[IBIS VER]   5.0
[File Name]   f28p551pm.ibs
[File Rev]   1.0
[Date]   August 04, 2025
[Source]   File originated at Texas Instruments
[Copyright]   (c) 2012, Texas Instruments Inc.
[Component]   f28p551pm
[Manufacturer]  Texas Instruments
[Package]
| Variable   Typ   Min   Max
R_pkg  2.56E-01  1.11E-01  3.13E-01
L_pkg  6.62E-09  4.95E-09  7.77E-09
C_pkg  9.34E-15  7.88E-15  1.08E-14
[Pin]   signal_name   model_name   R_pin   L_pin   C_pin
   1   GPIO29   BCF3385DSHYPBFZ_LC  2.96E-01  7.53E-09  1.05E-14
   2   A16,B16,C16,GPIO28   BCF3385DSHYPBFZ_LC  2.80E-01  7.22E-09  1.01E-14
   3   XRSn   BQ0491FS_USF  2.66E-01  6.93E-09  9.76E-15
   4   VDD   NC  1.47E-01  5.55E-09  8.58E-15
   5   VSS   NC  1.44E-01  5.38E-09  8.29E-15
   6   A6,D14,E14,GPIO228   BCF3385DSHYPBFZ_LC_USF  2.71E-01  6.53E-09  8.98E-15
   7   B2,C6,E12,GPIO226   BCF3385DSHYPBFZ_LC_USF  2.62E-01  6.29E-09  8.63E-15
   8   A3,B3,C5,GPIO242,PGA2_INP   BCF3385DSHYPBFZ_LC_USF  2.57E-01  6.10E-09  8.33E-15
   9   A2,B6,C9,GPIO224,PGA1_INP   BCF3385DSHYPBFZ_LC  2.56E-01  6.08E-09  8.32E-15
   10   A15,B9,C7,PGA1_INM   ICF33SHYPB_LC  2.55E-01  6.22E-09  8.59E-15
   11   A14,B14,C4,PGA1_OUT   ICF33SHYPB_LC  2.54E-01  6.36E-09  8.85E-15
   12   A11,B10,C0,PGA2_OUT   ICF33SHYPB_LC  2.57E-01  6.53E-09  9.14E-15
   13   A5,B12,C2,PGA2_INM   ICF33SHYPB_LC  2.63E-01  6.74E-09  9.46E-15
   14   A1,B7,D11,DACB_OUT   ICF33SHYPB_LC  2.74E-01  7.01E-09  9.82E-15
   15   A0,B15,C15,DACA_OUT   ICF33SHYPB_LC  2.90E-01  7.32E-09  1.02E-14
   16   D20,E20,VREFHI   ICF33SHYPB_LC  1.21E-01  5.73E-09  9.21E-15
   17   A13,B13,C13,D13,E13,VREFLO   ICF33SHYPB_LC  1.23E-01  5.83E-09  9.36E-15
   18   A12,C1,E11,PGA3_INP   ICF33SHYPB_LC  3.02E-01  7.51E-09  1.04E-14
   19   A7,B30,C3,D12,E30,PGA3_INM   ICF33SHYPB_LC  2.94E-01  7.28E-09  1.01E-14
   20   A8,B0,C11,PGA3_OUT   ICF33SHYPB_LC  2.86E-01  7.05E-09  9.76E-15
   21   VSSA   ICF33SHYPB_LC  1.15E-01  5.14E-09  8.18E-15
   22   VDDA   ICF33SHYPB_LC  1.11E-01  4.95E-09  7.88E-15
   23   A4,B8,C14   ICF33SHYPB_LC  2.82E-01  6.56E-09  8.90E-15
   24   A9,B4,C8,GPIO227,GPIO236   BCF3385DSHYPBFZ_LC  2.91E-01  6.50E-09  8.69E-15
   25   A10,B1,C10,GPIO230   BCF3385DSHYPBFZ_LC  2.81E-01  6.40E-09  8.61E-15
   26   VSS   NC  1.55E-01  5.25E-09  7.93E-15
   27   A17,B17,C17,CMP1_DACL,GPIO20   BCF3385DSHYPBFZ_LC  2.83E-01  6.72E-09  9.18E-15
   28   A18,B18,C18,GPIO21   BCF3385DSHYPBFZ_LC  2.78E-01  6.81E-09  9.42E-15
   29   A19,B19,C19,GPIO13   BCF3385DSHYPBFZ_LC  2.77E-01  6.96E-09  9.69E-15
   30   A20,B20,C20,GPIO12   BCF3385DSHYPBFZ_LC  2.81E-01  7.15E-09  1.00E-14
   31   A24,D0,E0,GPIO11   BCF3385DSHYPBFZ_LC  2.87E-01  7.36E-09  1.03E-14
   32   B24,D1,E1,GPIO33   BCF3385DSHYPBFZ_LC  3.13E-01  7.77E-09  1.08E-14
   33   C24,D2,E2,GPIO16   BCF3385DSHYPBFZ_LC  3.04E-01  7.61E-09  1.06E-14
   34   A25,D3,E3,GPIO17   BCF3385DSHYPBFZ_LC  2.84E-01  7.26E-09  1.02E-14
   35   B25,D4,E4,GPIO24   BCF3385DSHYPBFZ_LC  2.73E-01  6.99E-09  9.81E-15
   36   TCK   BCF3355DSHYPBFZ_TMS_USF  2.79E-01  6.92E-09  9.59E-15
   37   GPIO37/TDO   BCPF335585DSHYPBFZ  2.68E-01  6.65E-09  9.23E-15
   38   TMS   BCF3355DSHYPBFZ_TMS  2.62E-01  6.44E-09  8.91E-15
   39   GPIO35/TDI   BCF3385DSHYPBFZ_LC  2.60E-01  6.27E-09  8.62E-15
   40   GPIO32   BQ3320HYPBFZ_3VSBLK_5FS_LC  2.62E-01  6.14E-09  8.36E-15
   41   GPIO18,X2   BCF3385DSHYPBFZ_LC  2.61E-01  6.14E-09  8.36E-15
   42   GPIO19,X1   BCPF335585DSHYPBFZ  2.61E-01  6.29E-09  8.63E-15
   43   VDDIO   NC  2.71E-01  6.54E-09  8.98E-15
   44   VDD   NC  1.46E-01  5.39E-09  8.30E-15
   45   VSS   NC  1.14E-01  5.21E-09  8.33E-15
   46   VREGENZ   IQ0440FS_VREGENZ_USF  2.75E-01  7.02E-09  9.83E-15
   47   GPIO8   BCF3385DSHYPBFZ_LC  2.87E-01  7.29E-09  1.02E-14
   48   GPIO4   BCF3385DSHYPBFZ_LC  3.00E-01  7.57E-09  1.06E-14
   49   GPIO3  BQ3320HYPBFZ_3VSBLK_5FS_LC  3.07E-01  7.72E-09  1.08E-14
   50   GPIO2  BQ3320HYPBFZ_3VSBLK_5FS_LC  3.00E-01  7.50E-09  1.04E-14
   51   GPIO1   BCF3385DSHYPBFZ_LC  2.92E-01  7.27E-09  1.01E-14
   52   GPIO0   BCF3385DSHYPBFZ_LC  2.84E-01  7.02E-09  9.74E-15
   53   GPIO40   BCF3385DSHYPBFZ_LC  2.79E-01  6.82E-09  9.43E-15
   54   GPIO23   BCF3385DSHYPBFZ_LC  2.78E-01  6.67E-09  9.15E-15
   55   GPIO41   BCF3385DSHYPBFZ_LC  2.81E-01  6.54E-09  8.89E-15
   56   GPIO22   BCF3385DSHYPBFZ_LC  2.85E-01  6.44E-09  8.64E-15
   57   GPIO7   BCF3385DSHYPBFZ_LC  3.01E-01  6.60E-09  8.76E-15
   58   VSS   NC  1.61E-01  5.31E-09  7.98E-15
   59   VDD   NC  1.65E-01  5.50E-09  8.28E-15
   60   VDDIO   NC  3.09E-01  7.13E-09  9.66E-15
   61   GPIO5   BCF3385DSHYPBFZ_LC  2.93E-01  7.12E-09  9.81E-15
   62   GPIO9  BQ3320HYPBFZ_3VSBLK_5FS_LC  3.05E-01  7.40E-09  1.02E-14
   63   GPIO10   BCF3385DSHYPBFZ_LC_USF  3.05E-01  7.54E-09  1.05E-14
   64   GPIO6   BCF3385DSHYPBFZ_LC_USF  3.10E-01  7.74E-09  1.08E-14
| End of package information
|   Component BQ0491FS_USF
[Component]   BQ0491FS_USF
[Manufacturer]   Texas Instruments
[Package]
|  variable   typ   min   max
R_pkg   0   0   0
L_pkg   0   0   0
C_pkg   0   0   0
[Pin]   signal_name   model_name   R_pin   L_pin   C_pin
VSS   VSS   GND
VDDS   VDDS   POWER
PAD   PAD   BQ0491FS_USF
[Model Selector] BQ0491FS_USF
WK_PU_ON_WITH_RX_3P3  Cell operated at 3.3(nom)
|WK_PU_ON_WITH_RX_3P3; WEAK_PULLUP_ON_WITH_RX
OPEN_DRAIN_MODE_3P3  Cell operated at 3.3(nom)
|   Component BCPF335585DSHYPBFZ
[Component]   BCPF335585DSHYPBFZ
[Manufacturer]   Texas Instruments
[Package]
|  variable   typ   min   max
R_pkg   0   0   0
L_pkg   0   0   0
C_pkg   0   0   0
[Pin]   signal_name   model_name   R_pin   L_pin   C_pin
VSS   VSS   GND
VDDS   VDDS   POWER
PAD   PAD   BCPF335585DSHYPBFZ
[Model Selector] BCPF335585DSHYPBFZ
BCPF_WK_PU_ON_3P3  Cell operated at 3.3(nom)
|BCPF_WK_PU_ON_3P3; WEAK_PULLUP_ON
BCPF_DRIVER_MODE_4MA_3P3  Cell operated at 3.3(nom)
|BCPF_DRIVER_MODE_4MA_3P3
BCPF_DRIVER_MODE_2MA_3P3  Cell operated at 3.3(nom)
|BCPF_DRIVER_MODE_2MA_3P3
BCPF_WK_PD_ON_3P3  Cell operated at 3.3(nom)
|   Component ICF33SHYPB_LC
[Component]   ICF33SHYPB_LC
[Manufacturer]   Texas Instruments
[Package]
|  variable   typ   min   max
R_pkg   0   0   0
L_pkg   0   0   0
C_pkg   0   0   0
[Pin]   signal_name   model_name   R_pin   L_pin   C_pin
VSS   VSS   GND
VDDS   VDDS   POWER
PAD   PAD   ICF33SHYPB_LC
[Model Selector] ICF33SHYPB_LC
ICF_RECEIVER_MODE_3P3  Cell operated at 3.3(nom)
|ICF_RECEIVER_MODE_3P3; RECEIVER_MODE
ICF_WK_PU_ON_3P3  Cell operated at 3.3(nom)
|ICF_WK_PU_ON_3P3; WEAK_PULLUP_ON
ICF_WK_PD_ON_3P3  Cell operated at 3.3(nom)
|   Component BCF3385DSHYPBFZ_LC_USF
[Component]   BCF3385DSHYPBFZ_LC_USF
[Manufacturer]   Texas Instruments
[Package]
|  variable   typ   min   max
R_pkg   0   0   0
L_pkg   0   0   0
C_pkg   0   0   0
[Pin]   signal_name   model_name   R_pin   L_pin   C_pin
VSS   VSS   GND
VDDS   VDDS   POWER
PAD   PAD   BCF3385DSHYPBFZ_LC_USF
[Model Selector] BCF3385DSHYPBFZ_LC_USF
BCF_WK_PU_ON_3P3  Cell operated at 3.3(nom)
|BCF_WK_PU_ON_3P3; WEAK_PULLUP_ON
BCF_WK_PD_ON_3P3  Cell operated at 3.3(nom)
|BCF_WK_PD_ON_3P3; WEAK_PULLDOWN_ON
BCF_DRIVER_MODE_3P3  Cell operated at 3.3(nom)
|BCF_DRIVER_MODE_3P3
BCF_RECEIVER_MODE_3P3  Cell operated at 3.3(nom)
|   Component BCF3355DSHYPBFZ_TMS_USF
[Component]   BCF3355DSHYPBFZ_TMS_USF
[Manufacturer]   Texas Instruments
[Package]
|  variable   typ   min   max
R_pkg   0   0   0
L_pkg   0   0   0
C_pkg   0   0   0
[Pin]   signal_name   model_name   R_pin   L_pin   C_pin
VSS   VSS   GND
VDDS   VDDS   POWER
PAD   PAD   BCF3355DSHYPBFZ_TMS_USF
[Model Selector] BCF3355DSHYPBFZ_TMS_USF
TMS_WK_PU_ON_3P3  Cell operated at 3.3(nom)
|TMS_WK_PU_ON_3P3; WEAK_PULLUP_ON
TMS_DRIVER_3P3  Cell operated at 3.3(nom)
|TMS_DRIVER_3P3
TMS_WK_PD_ON_3P3  Cell operated at 3.3(nom)
|   Component BCF3385DSHYPBFZ_LC
[Component]   BCF3385DSHYPBFZ_LC
[Manufacturer]   Texas Instruments
[Package]
|  variable   typ   min   max
R_pkg   0   0   0
L_pkg   0   0   0
C_pkg   0   0   0
[Pin]   signal_name   model_name   R_pin   L_pin   C_pin
VSS   VSS   GND
VDDS   VDDS   POWER
PAD   PAD   BCF3385DSHYPBFZ_LC
[Model Selector] BCF3385DSHYPBFZ_LC
BCF_WK_PU_ON_3P3  Cell operated at 3.3(nom)
|BCF_WK_PU_ON_3P3; WEAK_PULLUP_ON
BCF_WK_PD_ON_3P3  Cell operated at 3.3(nom)
|BCF_WK_PD_ON_3P3; WEAK_PULLDOWN_ON
BCF_DRIVER_MODE_3P3  Cell operated at 3.3(nom)
|BCF_DRIVER_MODE_3P3
BCF_RECEIVER_MODE_3P3  Cell operated at 3.3(nom)
|BCF_RECEIVER_MODE_3P3; RECEIVER_MODE
|   Component IQ0440FS_VREGENZ_USF
[Component]   IQ0440FS_VREGENZ_USF
[Manufacturer]   Texas Instruments
[Package]
|  variable   typ   min   max
R_pkg   0   0   0
L_pkg   0   0   0
C_pkg   0   0   0
[Pin]   signal_name   model_name   R_pin   L_pin   C_pin
VSS   VSS   GND
VDDS   VDDS   POWER
PAD   PAD   IQ0440FS_VREGENZ_USF
[Model Selector] IQ0440FS_VREGENZ_USF
VREGENZ_WK_PD_ON_3P3  Cell operated at 3.3(nom)
|VREGENZ_WK_PD_ON_3P3; WEAK_PULLDOWN_ON
VREGENZ_WK_PD_OFF_3P3  Cell operated at 3.3(nom)
|   Component BCF3355DSHYPBFZ_TMS
[Component]   BCF3355DSHYPBFZ_TMS
[Manufacturer]   Texas Instruments
[Package]
|  variable   typ   min   max
R_pkg   0   0   0
L_pkg   0   0   0
C_pkg   0   0   0
[Pin]   signal_name   model_name   R_pin   L_pin   C_pin
VSS   VSS   GND
VDDS   VDDS   POWER
PAD   PAD   BCF3355DSHYPBFZ_TMS
[Model Selector] BCF3355DSHYPBFZ_TMS
TMS_WK_PU_ON_3P3  Cell operated at 3.3(nom)
|TMS_WK_PU_ON_3P3; WEAK_PULLUP_ON
TMS_DRIVER_3P3  Cell operated at 3.3(nom)
|TMS_DRIVER_3P3
TMS_WK_PD_ON_3P3  Cell operated at 3.3(nom)
|TMS_WK_PD_ON_3P3; WEAK_PULLDOWN_ON
|   Component BQ3320HYPBFZ_3VSBLK_5FS_LC
[Component] BQ3320HYPBFZ_3VSBLK_5FS_LC
[Manufacturer] Texas Instruments
[Package]
| variable   typ   min   max
R_pkg   0.0   0.0   0.0
L_pkg   0.0H   0.0H   0.0H
C_pkg   0.0F   0.0F   0.0F
[Pin]  signal_name   model_name   R_pin   L_pin   C_pin
PAD   PAD   BQ3320HYPBFZ_3VSBLK_5FS_LC
VDDS   VDDS   Power
VSS   VSS   Gnd
A   A   NC
GZ   GZ   NC
[Model Selector] BQ3320HYPBFZ_3VSBLK_5FS_LC
BQ3320HYPBFZ_3VSBLK_5FS_LC_M0_D0 I/O model with Mode = 0 and Drive = 0
BQ3320HYPBFZ_3VSBLK_5FS_LC_M0_D1 I/O model with Mode = 0 and Drive = 1
BQ3320HYPBFZ_3VSBLK_5FS_LC_M1_D0 I/O model with Mode = 1 and Drive = 0
BQ3320HYPBFZ_3VSBLK_5FS_LC_M1_D1 I/O model with Mode = 1 and Drive = 1
BQ3320HYPBFZ_3VSBLK_5FS_LC_PDON I/O model with Pulldown on PI=0 PSEL=0
BQ3320HYPBFZ_3VSBLK_5FS_LC_PUON I/O model with Pullup on PI=0 PSEL=0
| Models and submodels in the file (24): WK_PU_ON_WITH_RX_3P3 (Input), OPEN_DRAIN_MODE_3P3 (I/O_open_drain), BCPF_WK_PU_ON_3P3 (Input), BCPF_DRIVER_MODE_4MA_3P3 (I/O), BCPF_DRIVER_MODE_2MA_3P3 (I/O), BCPF_WK_PD_ON_3P3 (Input), ICF_RECEIVER_MODE_3P3 (Input), ICF_WK_PU_ON_3P3 (Input), ICF_WK_PD_ON_3P3 (Input), BCF_WK_PU_ON_3P3 (Input), BCF_WK_PD_ON_3P3 (Input), BCF_DRIVER_MODE_3P3 (I/O), BCF_RECEIVER_MODE_3P3 (Input), TMS_WK_PU_ON_3P3 (Input), TMS_DRIVER_3P3 (I/O), TMS_WK_PD_ON_3P3 (Input), VREGENZ_WK_PD_ON_3P3 (Input), VREGENZ_WK_PD_OFF_3P3 (Input), BQ3320HYPBFZ_3VSBLK_5FS_LC_M0_D0 (I/O), BQ3320HYPBFZ_3VSBLK_5FS_LC_M0_D1 (I/O), BQ3320HYPBFZ_3VSBLK_5FS_LC_M1_D0 (I/O), BQ3320HYPBFZ_3VSBLK_5FS_LC_M1_D1 (I/O), BQ3320HYPBFZ_3VSBLK_5FS_LC_PDON (Input), BQ3320HYPBFZ_3VSBLK_5FS_LC_PUON (Input)
